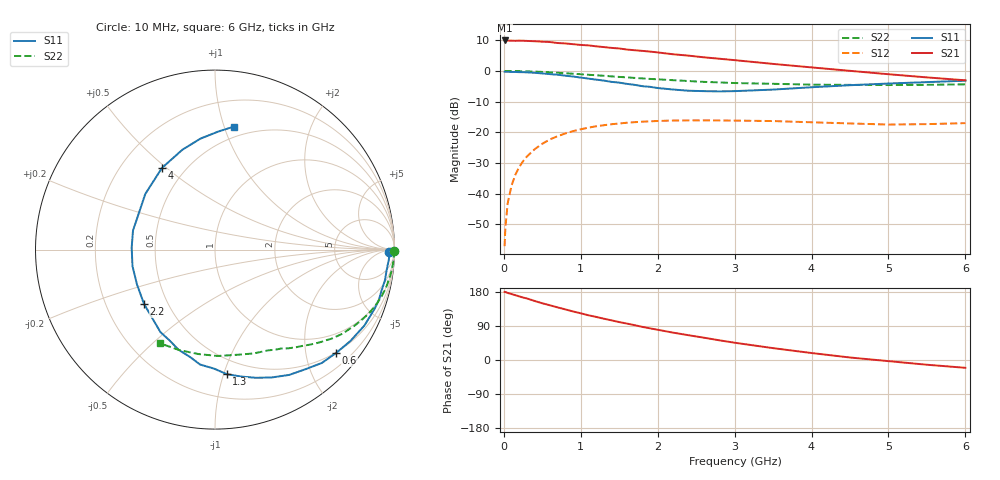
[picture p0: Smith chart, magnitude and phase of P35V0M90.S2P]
! SIEMENS Small Signal Semiconductors
! BFP181
! Si NPN RF Bipolar Junction Transistor in SOT143
! VCE = 5 V  IC = 0.9 mA
! Common Emitter S-Parameters:  March  1996
# GHz  S  MA  R  50
!  f  S11  S21  S12  S22
! GHz  MAG  ANG  MAG  ANG  MAG  ANG  MAG  ANG
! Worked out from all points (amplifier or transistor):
!   36 points, 10 MHz to 6 GHz, reference 50 ohm
!   highest |S21| = 9.9 dB at 10 MHz (marker M1)
!   |S21| within 3 dB of that: start of sweep to 1.616 GHz
!   unconditionally stable (mu >= 1): 3.318 GHz to end of sweep
!   at 250 MHz: K = 0.09, MSG = 19.6 dB, |S12| = -29.4 dB
!   at 1.4 GHz: K = 0.48, MSG = 12.4 dB, |S12| = -17.3 dB
!   at 6 GHz: K = 1.31, MAG = 3.7 dB, |S12| = -17.0 dB
!   S11 on the Smith chart (normalised r, x): 10 MHz: 55, -25; 600 MHz: 0.49, -2.64; 1.3 GHz: 0.38, -1.02; 2.2 GHz: 0.37, -0.30; 4 GHz: 0.37, +0.48; 6 GHz: 0.41, +1.08
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0.01  0.9704 -0.8  3.137 179.6  0.0014 89.8  0.9984 -0.3
0.02  0.9718 -1.4  3.129 179.4  0.0028 91.6  0.9952 -0.6
0.05  0.97 -3.3  3.121 177.0  0.007 90.8  0.9968 -1.7
0.1  0.9629 -7.1  3.114 174.1  0.0136 85.4  0.9963 -3.2
0.15  0.9622 -10.2  3.096 171.0  0.0205 82.8  0.994 -4.8
0.3  0.9485 -20.3  3.082 162.4  0.0404 76.2  0.9841 -9.5
0.4  0.934 -26.9  3.049 155.8  0.053 72.2  0.9761 -12.6
0.6  0.8874 -40.4  2.958 144.3  0.0768 63.3  0.9505 -18.5
0.8  0.8361 -52.8  2.805 133.5  0.096 55.4  0.9182 -23.9
1.1  0.7502 -72.2  2.607 118.0  0.1194 44.3  0.8662 -31.1
1.3  0.697 -84.6  2.447 109.0  0.1306 38.0  0.8334 -35.4
1.5  0.6457 -97.4  2.324 100.1  0.1392 32.5  0.7989 -39.2
1.8  0.565 -116.9  2.122 87.4  0.1491 25.5  0.7563 -44.1
2.2  0.4981 -142.5  1.869 72.2  0.1558 17.0  0.7071 -50.3
2.4  0.4762 -155.9  1.776 65.4  0.1565 13.4  0.6852 -53.4
2.8  0.4644 178.6  1.582 52.0  0.1564 7.8  0.6508 -59.0
3  0.4691 166.9  1.499 45.6  0.1553 5.0  0.6354 -62.0
3.5  0.4969 141.4  1.302 31.3  0.1527 0.3  0.6173 -69.6
4  0.5426 123.0  1.142 18.4  0.1459 -2.7  0.5983 -78.5
4.5  0.5857 108.0  1.004 6.6  0.1396 -4.6  0.5929 -88.6
5.5  0.6576 88.5  0.785 -12.5  0.1361 -1.3  0.5942 -109.5
6  0.6937 81.2  0.704 -20.6  0.1412 0.1  0.6051 -120.3
